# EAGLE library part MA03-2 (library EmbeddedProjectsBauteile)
PIN HEADER 2x3 polig
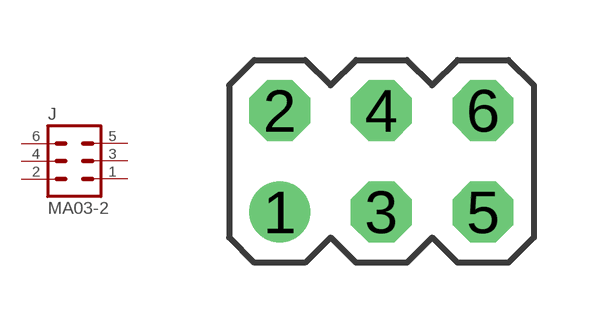
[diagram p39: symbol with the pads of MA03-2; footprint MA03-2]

Designator prefix J

## MA03-2 (EP: 400263)  [MA03-2]
1  1  pas
2  2  pas
3  3  pas
4  4  pas
5  5  pas
6  6  pas

## Footprint MA03-2 (pad centres in mm)
drill 1.016: 1 -2.54,-1.27
drill 1.016 octagon: 2 -2.54,1.27; 3 0,-1.27; 4 0,1.27; 5 2.54,-1.27; 6 2.54,1.27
